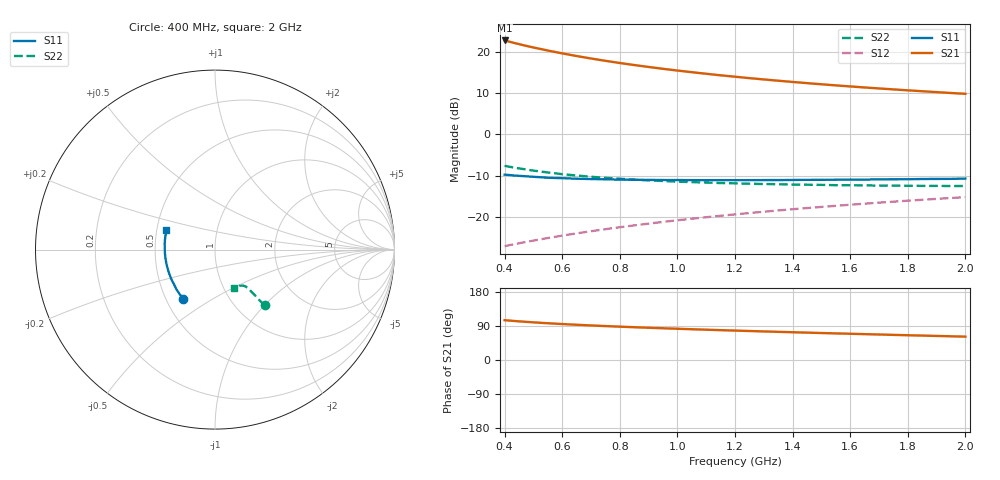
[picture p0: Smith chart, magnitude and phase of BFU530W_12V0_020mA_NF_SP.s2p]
! Filename:  P:\Prog\Test\Noise\ATS_data\Testdata_Net\06 Compressed Noise after Statistics\BFU530W_APM2013_09_A05_12p0V_020mA_NF_CM01_D.sf
! Date/Time: Tue 26/Mar/2013 18:06:01
! BFU530W_APM2013_09_A05_12p0V_1to25mA_NF_CM01_Bias8_R.sf
! Noise Parameter Data File
! BFU530W_APM2013_09_A05_12p0V_1to25mA_NF_CM01
! Date/time: Thu Mar 21 22:54:15 2013
! VAR V_out= 12.000000
! VAR I_out= 19.990000
! VAR V_in= 0.772900
! VAR I_in= 0.184250
! Device data file deembeded for feedlines and parallel
! Original file: \06 Compressed Noise after Statistics\BFU530W_APM2013_09_A05_12p0V_020mA_NF_CM01_R.sf
! Feed-files: PR019V01_070313_Feed1.s2p, PR019V01_070313_Feed2.s2p
! Parallel-file: PR019V01_070313_Par.s2p
# MHz S MA R 50
!  Freq-MHz  S11-mag  S11-arg  S21-mag  S21-arg  S12-mag  S12-arg  S22-mag  S22-arg
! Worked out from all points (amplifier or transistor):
!   37 points, 400 MHz to 2 GHz, reference 50 ohm
!   highest |S21| = 22.7 dB at 400 MHz (marker M1)
!   |S21| within 3 dB of that: start of sweep to 591.1 MHz
!   unconditionally stable (mu >= 1): 1.161 GHz to end of sweep
!   at 500 MHz: K = 0.85, MSG = 23.3 dB, |S12| = -25.7 dB
!   at 1.1 GHz: K = 1.00, MSG = 17.3 dB, |S12| = -20.0 dB
!   at 2 GHz: K = 1.01, MAG = 11.9 dB, |S12| = -15.2 dB
!   lowest NFmin = 1.07 dB at 420 MHz
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400  0.3263 -122.5  13.66 105.0  0.04452 64.8  0.4166 -48.1
420  0.3218 -125.3  13.1 103.8  0.04603 65.0  0.4046 -48.3
433  0.3184 -127.0  12.76 103.0  0.04698 65.1  0.397 -48.5
460  0.3139 -130.2  12.1 101.5  0.04902 65.5  0.3835 -48.6
500  0.3073 -134.9  11.23 99.4  0.05199 66.0  0.3649 -48.8
550  0.2991 -139.7  10.32 97.0  0.05586 66.6  0.3464 -48.9
600  0.2954 -144.2  9.537 94.9  0.05973 67.1  0.3304 -49.0
650  0.2912 -148.3  8.859 93.0  0.06356 67.5  0.3183 -49.0
700  0.2882 -152.1  8.268 91.2  0.06748 67.9  0.3075 -49.2
750  0.2862 -155.3  7.752 89.5  0.07143 68.3  0.298 -49.2
800  0.2838 -158.6  7.296 88.0  0.07544 68.5  0.2911 -49.5
850  0.2828 -161.5  6.893 86.5  0.07939 68.7  0.2836 -49.5
950  0.2806 -166.7  6.207 83.7  0.0875 69.1  0.2732 -50.0
1050  0.2799 -171.3  5.647 81.2  0.09556 69.2  0.265 -50.6
1150  0.2799 -175.7  5.18 78.8  0.1037 69.2  0.258 -51.3
1200  0.2795 -177.6  4.979 77.6  0.1079 69.2  0.2561 -51.9
1250  0.2798 -179.6  4.788 76.5  0.112 69.1  0.2531 -52.3
1350  0.2803 177.1  4.455 74.3  0.1203 68.9  0.2498 -53.4
1500  0.2823 172.1  4.035 71.2  0.1327 68.4  0.2451 -55.4
1650  0.2842 167.5  3.692 68.2  0.1452 67.9  0.2417 -57.4
1750  0.2865 164.9  3.499 66.3  0.1537 67.4  0.2404 -58.8
2000  0.2923 158.4  3.094 61.6  0.1745 66.1  0.2377 -63.0
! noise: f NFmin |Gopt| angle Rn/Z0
400  1.089  0.1879  -173.3  0.0914
460  1.082  0.2018  -170.3  0.0892
600  1.097  0.1962  -171  0.0917
800  1.133  0.211  -168.7  0.091
1000  1.155  0.2175  -165  0.0916
1200  1.211  0.2311  -163.2  0.09
1400  1.203  0.2543  -158.9  0.0892
1600  1.209  0.2634  -154.2  0.093
1800  1.258  0.2736  -152.9  0.0925
2000  1.26  0.2773  -149.4  0.1006
